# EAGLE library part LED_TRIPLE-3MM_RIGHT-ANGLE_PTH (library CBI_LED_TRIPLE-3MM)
CBI LED Triple-3mm, Right Angle, PTH E.g.: LUMEX SSF-LXH340LYGID
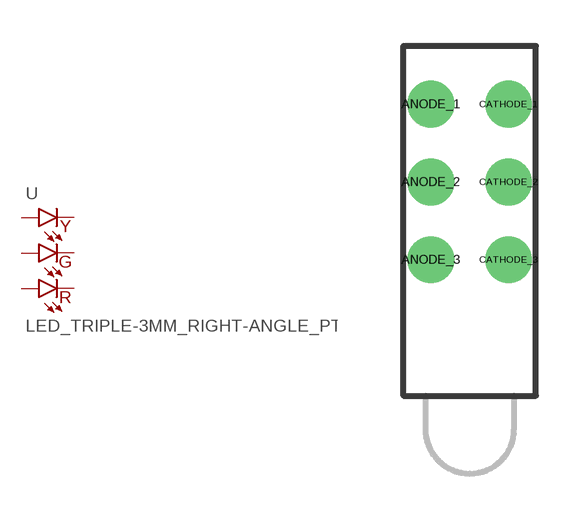
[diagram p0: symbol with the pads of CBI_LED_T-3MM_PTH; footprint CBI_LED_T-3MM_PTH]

Designator prefix -

## LED_TRIPLE-3MM_RIGHT-ANGLE_PTH_YELLOW_GREEN_RED (PROD_ID: DIO-19990; VALUE: Yellow Green Red)  [CBI_LED_T-3MM_PTH]
ANODE_1  YELLOW_ANODE  pas
ANODE_2  GREEN_ANODE  pas
ANODE_3  RED_ANODE  pas
CATHODE_1  YELLOW_CATHODE  pas
CATHODE_2  GREEN_CATHODE  pas
CATHODE_3  RED_CATHODE  pas

## Footprint CBI_LED_T-3MM_PTH (pad centres in mm)
CBI LED Triple-3mm E.g.: LUMEX SSF-LXH340LYGID
drill 0.889 pad 1.524: ANODE_1 -1.27,9.525; ANODE_2 -1.27,6.985; ANODE_3 -1.27,4.445; CATHODE_1 1.27,9.525; CATHODE_2 1.27,6.985; CATHODE_3 1.27,4.445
